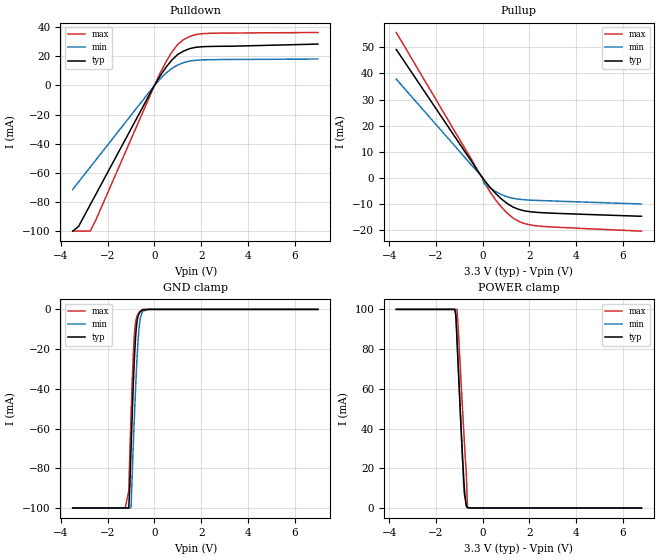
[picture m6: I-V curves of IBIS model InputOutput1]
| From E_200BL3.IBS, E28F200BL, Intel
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|********************Input Output Model 1**************************
[Model]   InputOutput1
Model_type   I/O
|   Model for DQ[0:14] pins.
Vinl = 0.8V
Vinh = 2.0V
|Variable   Typ   Min   Max
C_comp   9.61p   NA   11.6p
[Voltage Range]   3.3V   3.0V   3.6V
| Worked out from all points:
|   slope of the pulldown table from 0 to 0.495 V, typ, clamps not added: 39.8 ohm
|   slope of the pullup table from 0 to 0.495 V, typ, clamps not added: 92.9 ohm
|   GND clamp passes 1 mA (typ) near -0.59 V on its own axis
|   POWER clamp passes 1 mA (typ) near -0.69 V on its own axis
[Pulldown]
| [Pullup] and [Pulldown] IV curves include only the current through
| the channels of output driver transistors when outputs are enabled
| with OE# = VIL.  Although the output driver transistors have np and
| pn diodes inherently created by CMOS IC fabrication between the
| drain and bulk of n-channel and p-channel CMOS transistors,
| the current through these junction diodes is not included in
| [Pullup] or [Pulldown].  Instead that drain/bulk diode current is
| included in the [POWER_clamp] or [GND_clamp] sections, which are
| not dependent on the state of OE# or output data value.
|Voltage   I(typ)   I(min)   I(max)
-3.5V     -100mA     -71.39mA   -100mA
-3.25V    -96.81mA   -66.29mA   -100mA
-2.75V    -81.91mA   -56.09mA   -100mA
-2.5V     -74.46mA   -50.99mA   -92.02mA
-250mV    -7.275mA   -5.059mA   -9.23mA
250mV     6.697mA    4.573mA    8.667mA
750mV     17.51mA    11.72mA    22.95mA
1V        21.3mA     14.07mA    28.21mA
1.25V     23.59mA    15.65mA    31.56mA
1.75V     26.13mA    17.25mA    34.85mA
2.25V     26.71mA    17.6mA     35.72mA
7V        28.4mA     18.13mA    36.33mA
[GND_clamp]
| [POWER_clamp] and [GND_clamp] IV curves describe ESD protection
| circuits PLUS some np and pn diodes which exist between the
| drain and bulk of n-channel and p-channel CMOS transistors.
| These drain/bulk diodes are inherent in CMOS IC fabrication,
| and are visible on the node of the I/O pin at all times.
| Even the drain/bulk diodes of output driver [Pullup] and [Powerdown]
| transistors are included in [POWER_clamp] or [GND_clamp], because
| these diodes contribute to I/O pin current even when the
| chip outputs are tristated by OE# = VIH.
| For example, when V forced on the I/O pin is large, we are
| forward biasing the pn diode at the drain/bulk interface in the
| p-channel pullup transistor.  Similarly, when V forced on the
| I/O pin is sufficiently negative with respect to the substrate
| ground, we are forward biasing the np diode at the drain/bulk
| interface in the n-channel pulldown transistor.  The effects
| of these diodes are included in [POWER_clamp] or [GND_clamp].
|Voltage   I(typ)   I(min)   I(max)
-3.5V     -100mA     -100mA     -100mA
-1.25V    -100mA     -100mA     -100mA
-1.1V     -100mA     -100mA     -91.37mA
-1.05V    -87.98mA   -100mA     -71.58mA
-1V       -69.49mA   -99.32mA   -52.77mA
-900mV    -36.11mA   -66.6mA    -21.16mA
-850mV    -22.82mA   -51.75mA   -11.21mA
-800mV    -12.39mA   -37.71mA   -5.857mA
-700mV    -3.25mA    -15.39mA   -2.295mA
-600mV    -1.101mA   -4mA       -738.7uA
-250mV    0A         0A         0A
7V        0A         0A         0A
[Pullup]
| (Voltages for [Pullup] and [POWER_clamp] are specified with
| negative respect to Vcc.  Reference the IBIS documentation
| for more information regarding Vtable = Vcc - Voutput.
| This method keeps -Vds constant for the values in all three
| columns across a line of the table.
| [Pullup] and [Pulldown] IV curves include only the current through
| the channels of output driver transistors when outputs are enabled
| with OE# = VIL.  Although the output driver transistors have np and
| pn diodes inherently created by CMOS IC fabrication between the
| drain and bulk of n-channel and p-channel CMOS transistors,
| the current through these junction diodes is not included in
| [Pullup] or [Pulldown].  Instead that drain/bulk diode current is
| included in the [POWER_clamp] or [GND_clamp] sections, which are
| not dependent on the state of OE# or output data value.
|Voltage  I(typ)   I(min)   I(max)
-3.7V     49.17mA    37.82mA    55.67mA
-450mV    5.996mA    4.614mA    6.734mA
-200mV    2.555mA    2.26mA     2.458mA
0V        0A         0A         0A
50mV      -582.8uA   -1.966mA   -1.501mA
550mV     -5.876mA   -5.144mA   -8.312mA
800mV     -8.009mA   -6.324mA   -11.1mA
1.3V      -11.12mA   -7.766mA   -15.32mA
1.55V     -12.02mA   -8.126mA   -16.63mA
1.8V      -12.59mA   -8.332mA   -17.45mA
2.3V      -13.12mA   -8.56mA    -18.28mA
6.8V      -14.64mA   -9.94mA    -20.32mA
[POWER_clamp]
| (Voltages for [Pullup] and [POWER_clamp] are specified with
| negative respect to Vcc.  Reference the IBIS documentation
| for more information regarding Vtable = Vcc - Voutput.
| This method keeps -Vds constant for the values in all three
| columns across a line of the table.
| [POWER_clamp] and [GND_clamp] IV curves describe ESD protection
| circuits PLUS some np and pn diodes which exist between the
| drain and bulk of n-channel and p-channel CMOS transistors.
| These drain/bulk diodes are inherent in CMOS IC fabrication,
| and are visible on the node of the I/O pin at all times.
| Even the drain/bulk diodes of output driver [Pullup] and [Powerdown]
| transistors are included in [POWER_clamp] or [GND_clamp], because
| these diodes contribute to I/O pin current even when the
| chip outputs are tristated by OE# = VIH.
| For example, when V forced on the I/O pin is large, we are
| forward biasing the pn diode at the drain/bulk interface in the
| p-channel pullup transistor.  Similarly, when V forced on the
| I/O pin is sufficiently negative with respect to the substrate
| ground, we are forward biasing the np diode at the drain/bulk
| interface in the n-channel pulldown transistor.  The effects
| of these diodes are included in [POWER_clamp] or [GND_clamp].
|Voltage I(typ)   I(min)   I(max)
-3.7V     100mA      100mA      100mA
-1.2V     100mA      100mA      100mA
-1.15V    96.88mA    99.61mA    100mA
-1.1V     84.37mA    86.22mA    100mA
-1.05V    71.77mA    72.83mA    91.38mA
-900mV    34.29mA    33.22mA    57.82mA
-850mV    22.75mA    20.81mA    47mA
-800mV    12.63mA    7.246mA    36.38mA
-750mV    5.049mA    5.522mA    26.28mA
-700mV    1.276mA    491.9uA    17.04mA
-650mV    215.7uA    0A         0A
6.8V      0A         0A         0A
[Ramp]
| The DQ Ramp information is not provided at this time for the
| device but will be available in the future.  The table below
| is for the compatibility with some IBIS parsers.
| Variable   typ   min   max
 dV/dt_r   0V/0ns   0V/0ns   0V/0ns
 dV/dt_f   0V/0ns   0V/0ns   0V/0ns
